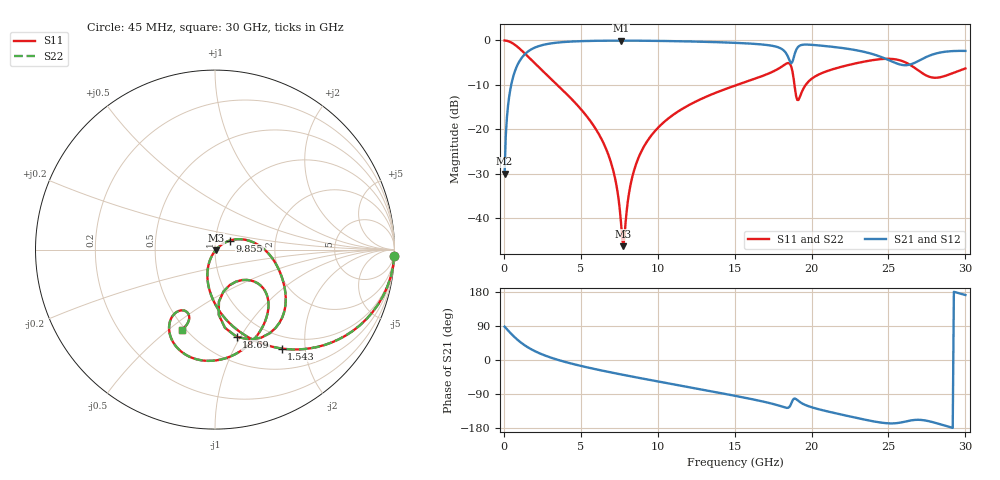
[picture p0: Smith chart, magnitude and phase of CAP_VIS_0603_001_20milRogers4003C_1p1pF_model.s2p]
! S-parameter model data by Modelithics Inc.  support@modelithics.com  813-866-6335  Tampa FL USA
! S-Parameter data specifications:
! Substrate: 20-mil Rogers 4003C, substrate thickness, H=0.508mm, Dielectric constant, Er=3.75
! PCB Mounting Pad Footprint: Pad width, PadW=0.90mm , Pad length, PadL=1.00mm , Pad gap, PadG (edge-to-edge)=1.00mm , Reference planes=3.0mm apart
! Created Wed Nov 18 13:17:44 2015
# hz S ma R 50
! 2 Port Network Data from SP1.SP block
! freq  magS11  angS11  magS21  angS21  magS12  angS12  magS22  angS22
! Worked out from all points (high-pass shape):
!   401 points, 45 MHz to 30 GHz, reference 50 ohm
!   highest |S21| = -0.05 dB at 7.609 GHz (marker M1); lowest = -30.0 dB at 45 MHz (marker M2)
!   |S21| within 3 dB of the highest: 1.378 GHz to 18.37 GHz (16.99 GHz wide, 172 % of centre); 18.91 GHz to 23.94 GHz (5.039 GHz wide, 23.5 % of centre)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
!   lowest |S11| = -46.3 dB at 7.758 GHz (marker M3), VSWR 1.01, Z = 50.4 - j0.315 ohm
!   |S11| at or under -10 dB: 3.466 GHz to 15.16 GHz (11.7 GHz wide, 126 % of centre); 18.89 GHz to 19.62 GHz (733.7 MHz wide, 3.81 % of centre)
!   |S22| runs from -46.3 to 0.0 dB; largest |S21 - S12| = 0
!   S11 on the Smith chart (normalised r, x): 45 MHz: 1, -56; 1.543 GHz: 0.80, -1.58; 9.855 GHz: 1.17, +0.12; 18.69 GHz: 0.74, -0.96; 30 GHz: 0.48, -0.56
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4.5e7  0.9995 -2.0  0.03151 88.0  0.03151 88.0  0.9995 -2.0
2.696625e8  0.9825 -12.1  0.1858 77.9  0.1858 77.9  0.9825 -12.1
4.94325e8  0.9444 -21.7  0.3282 68.3  0.3282 68.3  0.9444 -21.7
1.54275e9  0.6646 -56.0  0.7455 33.8  0.7455 33.8  0.6646 -56.0
2.965612e9  0.3827 -82.1  0.9209 7.5  0.9209 7.5  0.3827 -82.1
5.062462e9  0.1639 -104.9  0.9823 -16.2  0.9823 -16.2  0.1639 -104.9
6.859762e9  0.0478 -116.6  0.9938 -32.0  0.9938 -32.0  0.0478 -116.6
7.309088e9  0.02369 -114.3  0.9944 -35.6  0.9944 -35.6  0.02369 -114.3
7.608638e9  0.009041 -96.2  0.9945 -38.0  0.9945 -38.0  0.009041 -96.2
7.758412e9  0.004828 -40.3  0.9945 -39.2  0.9945 -39.2  0.004828 -40.3
8.507288e9  0.03663 36.9  0.9935 -45.1  0.9935 -45.1  0.03663 36.9
9.855262e9  0.097 31.2  0.9888 -55.4  0.9888 -55.4  0.097 31.2
1.007992e10  0.1066 29.8  0.9877 -57.1  0.9877 -57.1  0.1066 29.8
1.50225e10  0.31 -6.3  0.9397 -94.5  0.9397 -94.5  0.31 -6.3
1.8018e10  0.5012 -38.5  0.8098 -122.2  0.8098 -122.2  0.5012 -38.5
1.869199e10  0.5 -76.1  0.5541 -113.6  0.5541 -113.6  0.5 -76.1
1.914131e10  0.2136 -56.5  0.8509 -108.0  0.8509 -108.0  0.2136 -56.5
2.003996e10  0.3741 -40.4  0.8916 -125.1  0.8916 -125.1  0.3741 -40.4
2.266102e10  0.5417 -65.8  0.7895 -150.5  0.7895 -150.5  0.5417 -65.8
2.505742e10  0.6213 -97.2  0.5965 -167.2  0.5965 -167.2  0.6213 -97.2
2.752871e10  0.3975 -120.6  0.6594 -160.6  0.6594 -160.6  0.3975 -120.6
3e10  0.4838 -112.6  0.7617 171.5  0.7617 171.5  0.4838 -112.6
